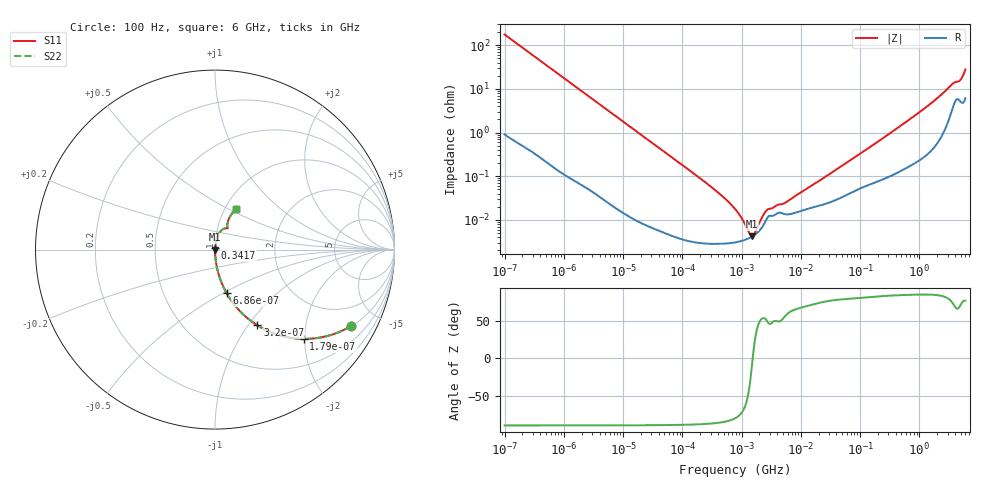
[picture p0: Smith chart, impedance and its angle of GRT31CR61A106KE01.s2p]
!Murata Part Number: GRT31CR61A106KE01
!These Parameters are Measured in Series Mode Connection
!Data Generated on Jun 19, 2026
!  o--ll--o
!Port1  Port2
!  o------o
!Operation Temp=25[degC], DC Bias Voltage=0[V]
!Freq. Start=100[Hz] Stop=6[GHz] 401[Steps]
# Hz S RI R 50
!Freq.(Hz) S11(Real) S11(Imag) S21(Real) S21(Imag) S12(Real) S12(Imag) S22(Real) S22(Imag)
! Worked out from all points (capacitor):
!   401 points, 100 Hz to 6 GHz, reference 50 ohm
!   read as one part in series: C = 9 uF near 109 Hz
!   lowest |Z| = 4.2 mohm at 1.516 MHz (marker M1)
!   series resonance near 1.54 MHz, so ESL is about 1.2 nH
!   S11 on the Smith chart (normalised r, x): 100 Hz: 1.02, -3.53; 179 Hz: 1.01, -1.98; 320 Hz: 1.01, -1.11; 686 Hz: 1.00, -0.52; 341.7 MHz: 1.00, +0.02; 6 GHz: 1.12, +0.54
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100  0.7559 -0.427  0.2441 0.427  0.2441 0.427  0.7559 -0.427
179  0.494 -0.4972  0.506 0.4972  0.506 0.4972  0.494 -0.4972
320  0.2357 -0.4215  0.7643 0.4215  0.7643 0.4215  0.2357 -0.4215
458  0.1319 -0.3354  0.8681 0.3354  0.8681 0.3354  0.1319 -0.3354
686  0.0642 -0.2422  0.9358 0.2422  0.9358 0.2422  0.0642 -0.2422
2008  0.00845 -0.0881  0.9916 0.0881  0.9916 0.0881  0.00845 -0.0881
6433  0.000991 -0.0279  0.999 0.0279  0.999 0.0279  0.000991 -0.0279
40335  7.64e-05 -0.00448  0.9999 0.00448  0.9999 0.00448  7.64e-05 -0.00448
330837  2.85e-05 -0.000525  1 0.000525  1 0.000525  2.85e-05 -0.000525
774597  3.05e-05 -0.000176  1 0.000176  1 0.000176  3.05e-05 -0.000176
1059725  3.37e-05 -9.1e-05  1 9.1e-05  1 9.1e-05  3.37e-05 -9.1e-05
1516199  4.18e-05 -3.7e-06  1 3.7e-06  1 3.7e-06  4.18e-05 -3.7e-06
1983483  5.61e-05 6.25e-05  0.9999 -6.25e-05  0.9999 -6.25e-05  5.61e-05 6.25e-05
2837864  0.00012 0.000131  0.9999 -0.000131  0.9999 -0.000131  0.00012 0.000131
5554849  0.000134 0.000211  0.9999 -0.000211  0.9999 -0.000211  0.000134 0.000211
1.555665e7  0.000191 0.000589  0.9998 -0.000589  0.9998 -0.000589  0.000191 0.000589
3.124326e8  0.00107 0.00935  0.9989 -0.00935  0.9989 -0.00935  0.00107 0.00935
3.417016e8  0.00114 0.0102  0.9989 -0.0102  0.9989 -0.0102  0.00114 0.0102
1.431855e9  0.00508 0.0417  0.9949 -0.0417  0.9949 -0.0417  0.00508 0.0417
3.505958e9  0.0427 0.1125  0.9573 -0.1125  0.9573 -0.1125  0.0427 0.1125
4.796499e9  0.0685 0.1269  0.9315 -0.1269  0.9315 -0.1269  0.0685 0.1269
6e9  0.1154 0.2263  0.8846 -0.2263  0.8846 -0.2263  0.1154 0.2263
